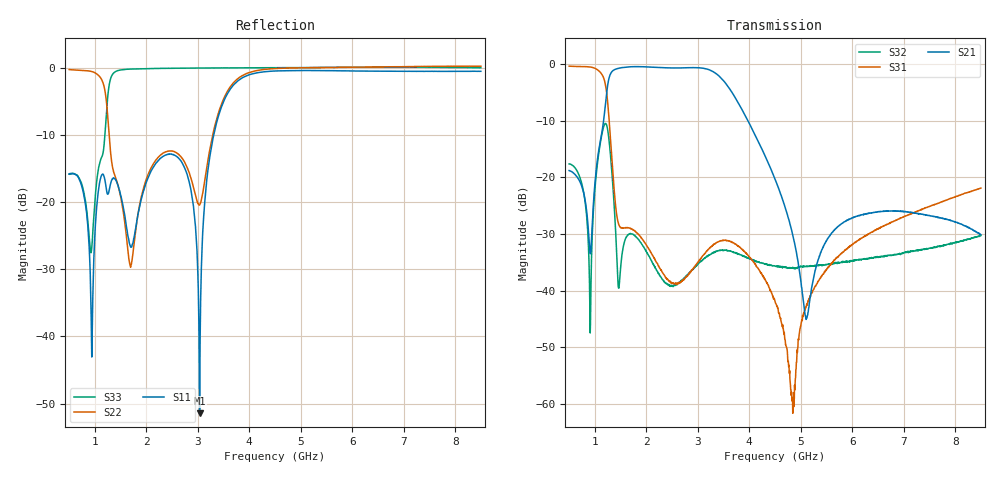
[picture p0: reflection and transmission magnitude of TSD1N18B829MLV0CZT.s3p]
# MHZ S RI R 50
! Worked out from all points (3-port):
!   1601 points, 500 MHz to 8.5 GHz, reference 50 ohm
!   strongest paths, dB at 500 MHz, 2.5 GHz, 4.5 GHz, 6.5 GHz, 8.5 GHz:
!     S21: -18.8, -0.7, -20.3, -26.1, -30.1
!     S31: -0.4, -38.6, -41.9, -29.1, -21.9
!     S32: -17.6, -39.2, -35.7, -34.2, -30.3
!   lowest |S11| = -51.4 dB at 3.035 GHz (marker M1), VSWR 1.01, Z = 50.1 - j0.255 ohm
!   |S11| at or under -10 dB: start of sweep to 3.311 GHz
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500  -0.1567 -0.0405  0.0994 0.0578  0.4696 -0.8359
     0.0993 0.0573  -0.3461 -0.9035  0.1193 -0.0541
     0.4705 -0.8357  0.1197 -0.0541  -0.1004 -0.1259
910  -0.000985 0.0297  0.00484 0.0206  -0.5707 -0.751
     0.00482 0.0206  -0.9403 0.0196  0.00289 -0.00292
     -0.5703 -0.7511  0.00293 -0.00303  -0.0182 -0.0412
1155  -0.1565 0.0393  -0.2094 0.1868  -0.7211 0.3087
      -0.2093 0.1876  -0.3488 0.6958  0.137 -0.2244
      -0.7218 0.3088  0.1374 -0.2237  0.1778 -0.1428
1470  -0.1033 -0.0708  0.4985 0.773  -0.0252 0.028
      0.4995 0.7735  -0.000222 0.1236  0.0105 0.0019
      -0.0254 0.0281  0.0105 0.00202  -0.0719 -0.953
2680  -0.157 -0.1245  0.5608 -0.7377  0.00141 0.012
      0.5585 -0.7382  -0.1431 -0.1606  -0.00218 -0.0118
      0.0014 0.0119  -0.0023 -0.012  -0.8749 -0.4662
3035  0.000851 -0.00254  0.1321 -0.9164  0.0119 0.0143
      0.1302 -0.9183  0.00149 -0.0951  -0.00736 -0.0159
      0.012 0.0144  -0.00738 -0.0161  -0.9174 -0.3828
3415  0.3751 -0.2558  -0.4293 -0.6553  0.0261 0.00778
      -0.4289 -0.6553  0.2904 -0.3793  -0.0205 -0.00924
      0.026 0.00786  -0.0206 -0.00948  -0.9476 -0.3049
4500  -0.3501 -0.8771  -0.0913 0.029  0.00642 -0.0048
      -0.092 0.0288  -0.4839 -0.8566  -0.00919 0.0137
      0.00644 -0.00485  -0.00899 0.0138  -0.9951 -0.0898
5110  -0.5793 -0.7552  -0.00354 -0.00474  -0.00153 0.00722
      -0.0034 -0.00454  -0.7201 -0.6914  -0.00566 0.0155
      -0.00177 0.00706  -0.00582 0.0153  -1.001 0.0324
8500  -0.9389 -0.0228  0.00489 -0.0308  0.0223 0.077
      0.0049 -0.0307  -1.024 -0.0446  0.00616 0.0296
      0.0225 0.0771  0.00602 0.03  -0.8983 0.4364
